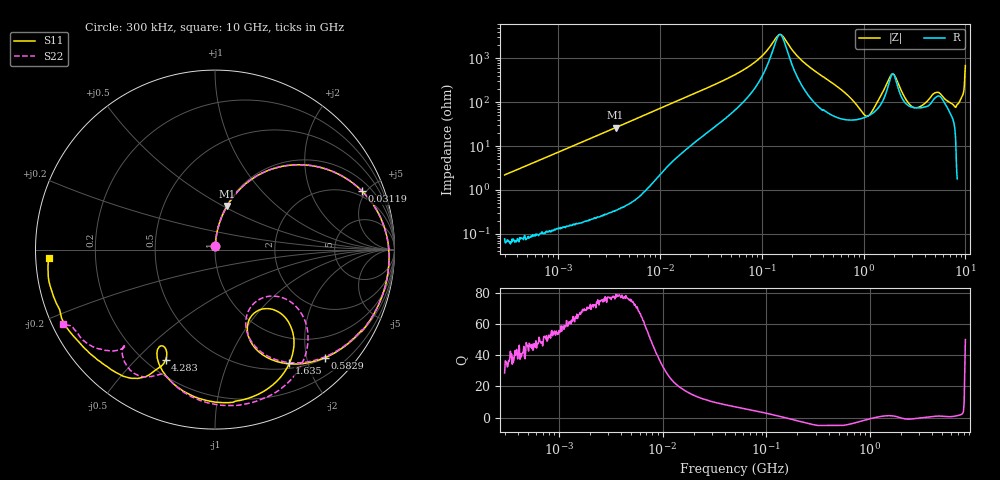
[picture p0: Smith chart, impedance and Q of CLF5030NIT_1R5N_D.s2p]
! S-Parameter Data Generated by TDK Corporation
! Copyright(C) 2019 TDK Corporation.
! All Rights Reserved.
! TDK P/N: CLF5030NIT-1R5N-D (Inductor)
! Property: L=1.5uH at 100kHz
! Size(LxWxT): 5.3x5x2.7mm
! Model Type: s2p (Touchstone File Format Version 1.0)
! Frequency: DC=Yes Start=0.3MHz Stop=10000MHz 802points Log-sweep
! Model Generated on May 10, 2019
! Port Assignments:
!  1 ---@@@--- 2
! Applicable Conditions:
!  Temperature = 25 degC
!  DC Bias Current = 0 A
!  Small Signal Operation
! Terms and conditions regarding TDK Simulation Models
! (1)This simulation model is being provided solely for informational purposes. Please refer to the specifications of the products in terms of detailed characteristics of such products.
! (2)In no event shall TDK Corporation of any of its subsidiaries be liable for any loss or damage arising, directly or indirectly,
!  From any information contained in this simulation model, including, but not limited to loss or damages arising from any inaccuracies, omissions or errors in connection with such information.
! (3)Any and all copyrights on this simulation model are owned by TDK Corporation.
!  Duplication or redistribution of this simulation model without prior written permission from TDK Corporation is prohibited.
! (4)This simulation model is subject to any modification or change without any prior notice.
! (5)Neither TDK Corporation nor any of its subsidiaries shall make any warranty, express or implied,
!  Including but not limited to the correctness, implied warranties of merchantability and fitness for a particular purpose with respect to this simulation models.
! (6)The use of this simulation model shall be deemed to have consented to the terms and conditions hereof.
# Hz S MA R 50
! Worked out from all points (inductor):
!   801 points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, 300 kHz to 10 GHz, reference 50 ohm
!   read as one part in series: L = 1.16 uH near 318.3 kHz
!   highest Q = 77.5 at 3.688 MHz (marker M1), where L = 1.14 uH
!   self-resonance near 151.5 MHz
!   S11 on the Smith chart (normalised r, x): 300 kHz: 1.00, +0.04; 31.19 MHz: 1.61, +4.71; 582.9 MHz: 0.51, -2.35; 1.635 GHz: 0.57, -1.70; 4.283 GHz: 0.27, -0.61; 10 GHz: 0.04, -0.02
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300000  0.022 86.9  0.9989 -1.2  0.9989 -1.2  0.02213 87.2
1713600  0.121 82.2  0.9909 -7.0  0.9909 -7.0  0.121 82.2
3688026  0.2527 74.5  0.9642 -14.8  0.9643 -14.8  0.2528 74.5
9671944  0.5628 53.7  0.8105 -34.6  0.8106 -34.6  0.5627 53.8
3.118733e7  0.8821 21.6  0.3907 -62.6  0.3907 -62.6  0.882 21.7
5.477226e7  0.941 10.4  0.2219 -70.6  0.222 -70.6  0.9411 10.5
9.444554e7  0.966 1.5  0.09836 -70.9  0.09838 -70.9  0.966 1.7
1.495617e8  0.9722 -5.9  0.02772 -10.9  0.02774 -10.9  0.9723 -5.7
3.126428e8  0.9559 -21.8  0.1618 57.4  0.1619 57.4  0.9564 -21.3
5.82867e8  0.8592 -44.4  0.366 35.2  0.3661 35.1  0.8604 -43.6
7.956093e8  0.7171 -60.7  0.5084 12.4  0.5084 12.4  0.7156 -59.9
1.024756e9  0.5036 -68.7  0.6076 -16.8  0.6076 -16.8  0.4851 -68.7
1.323741e9  0.479 -45.1  0.5459 -59.0  0.5456 -59.1  0.4301 -37.2
1.635219e9  0.7567 -56.8  0.2866 -91.4  0.2862 -91.5  0.7408 -45.8
1.767019e9  0.8188 -66.7  0.1879 -91.9  0.1875 -91.9  0.8169 -55.4
1.990462e9  0.8521 -82.3  0.1246 -58.8  0.1244 -58.7  0.8711 -70.5
2.720446e9  0.7445 -112.4  0.2734 -54.8  0.2731 -54.8  0.8219 -100.6
4.282745e9  0.6753 -114.1  0.2212 -127.9  0.2205 -127.7  0.7772 -115.4
5.849356e9  0.8657 -125.0  0.1124 -132.5  0.1128 -131.4  0.7405 -133.4
7.763894e9  0.9337 -152.3  0.08073 160.4  0.08286 160.8  0.8916 -145.5
9.105558e9  0.9416 -168.7  0.01851 127.7  0.0186 124.1  0.9142 -152.4
1e10  0.9284 -177.3  0.001358 11.3  0.001612 -10.5  0.9442 -154.1
